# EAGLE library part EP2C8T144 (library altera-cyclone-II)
EP2C8T144 Auto generated by make-symbol-device-package-bsdl.ulp Rev. 19 Tip: Use split-device-symbol.ulp to generate a Device with multiple small symbols! Read HELP. Source: EP2C8T144.BSD
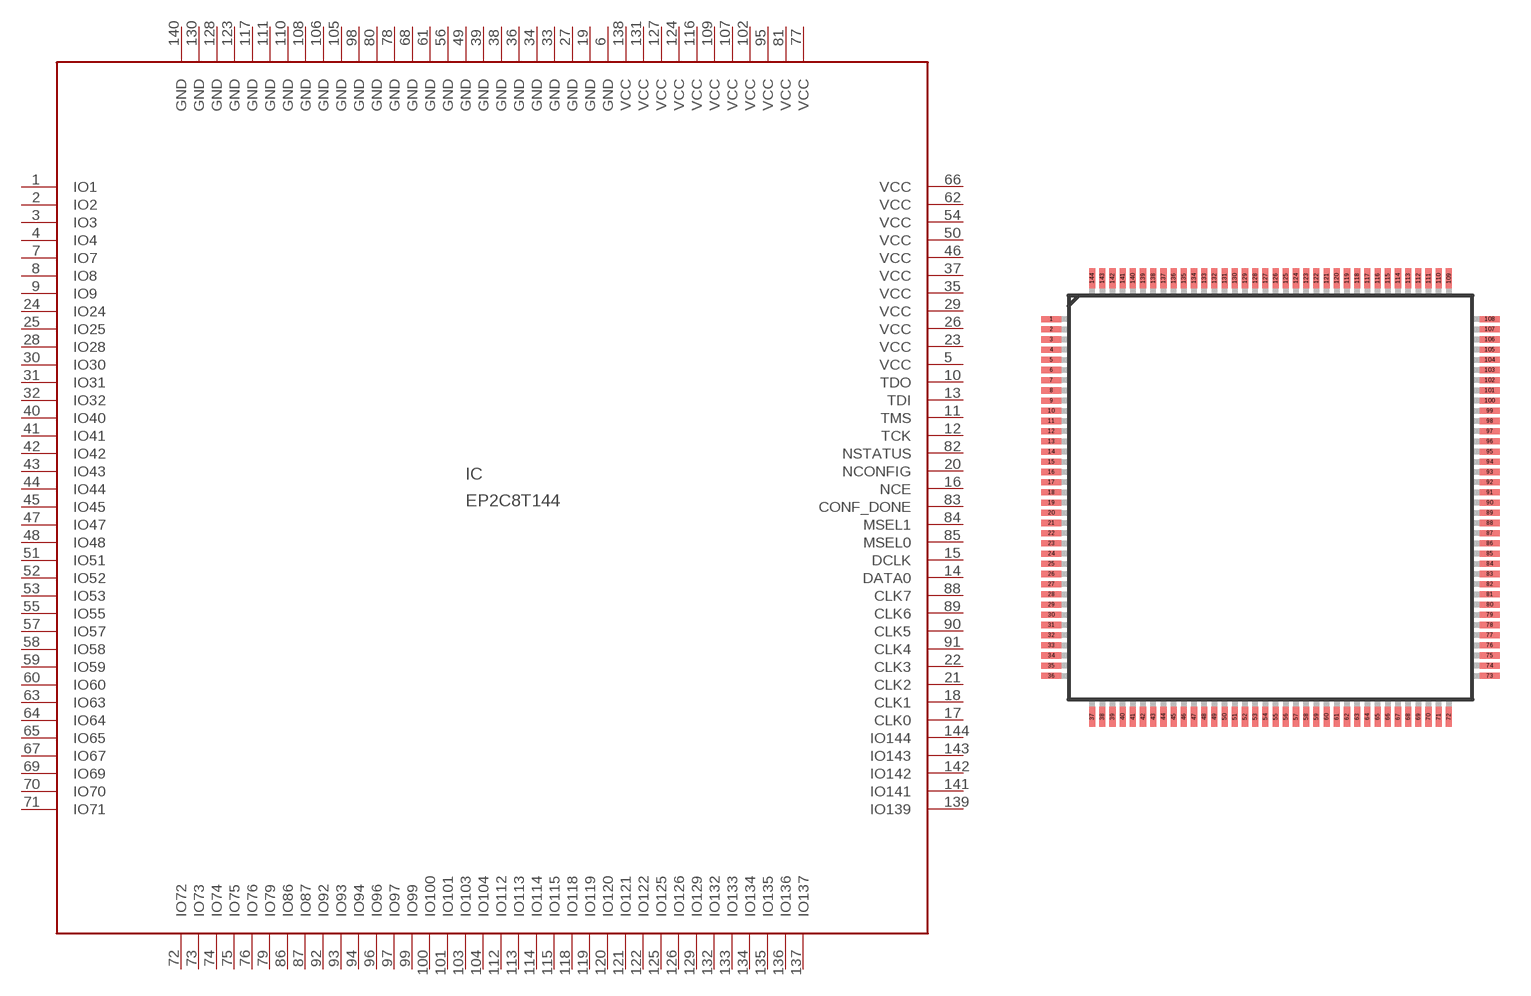
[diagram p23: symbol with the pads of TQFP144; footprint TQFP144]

Designator prefix IC

## EP2C8T144 (MPN: EP2C8T144C8N; OC_FARNELL: 1663192; OC_NEWARK: 51R0576)  [TQFP144]
1  IO1  out
2  IO2  out
3  IO3
4  IO4
5  VCC  pwr
6  GND  pwr
7  IO7
8  IO8
9  IO9
10  TDO  out
11  TMS  in
12  TCK  in
13  TDI  in
14  DATA0
15  DCLK
16  NCE  in
17  CLK0
18  CLK1
19  GND  pwr
20  NCONFIG  in
21  CLK2
22  CLK3
23  VCC  pwr
24  IO24
25  IO25
26  VCC  pwr
27  GND  pwr
28  IO28
29  VCC  pwr
30  IO30
31  IO31
32  IO32
33  GND  pwr
34  GND  pwr
35  VCC  pwr
36  GND  pwr
37  VCC  pwr
38  GND  pwr
39  GND  pwr
40  IO40
41  IO41
42  IO42
43  IO43
44  IO44
45  IO45
46  VCC  pwr
47  IO47
48  IO48
49  GND  pwr
50  VCC  pwr
51  IO51
52  IO52
53  IO53
54  VCC  pwr
55  IO55
56  GND  pwr
57  IO57
58  IO58
59  IO59
60  IO60
61  GND  pwr
62  VCC  pwr
63  IO63
64  IO64
65  IO65
66  VCC  pwr
67  IO67
68  GND  pwr
69  IO69
70  IO70
71  IO71
72  IO72
73  IO73
74  IO74
75  IO75
76  IO76
77  VCC  pwr
78  GND  pwr
79  IO79
80  GND  pwr
81  VCC  pwr
82  NSTATUS  in
83  CONF_DONE  in
84  MSEL1  in
85  MSEL0  in
86  IO86
87  IO87
88  CLK7
89  CLK6
90  CLK5
91  CLK4
92  IO92
93  IO93
94  IO94
95  VCC  pwr
96  IO96
97  IO97
98  GND  pwr
99  IO99
100  IO100
101  IO101
102  VCC  pwr
103  IO103
104  IO104
105  GND  pwr
106  GND  pwr
107  VCC  pwr
108  GND  pwr
109  VCC  pwr
110  GND  pwr
111  GND  pwr
112  IO112
113  IO113
114  IO114
115  IO115
116  VCC  pwr
117  GND  pwr
118  IO118
119  IO119
120  IO120
121  IO121
122  IO122
123  GND  pwr
124  VCC  pwr
125  IO125
126  IO126
127  VCC  pwr
128  GND  pwr
129  IO129
130  GND  pwr
131  VCC  pwr
132  IO132
133  IO133
134  IO134
135  IO135
136  IO136
137  IO137
138  VCC  pwr
139  IO139
140  GND  pwr
141  IO141
142  IO142
143  IO143
144  IO144

## Footprint TQFP144 (pad centres in mm)
TQFP144 Auto generated by make-symbol-device-package-bsdl.ulp Rev. 19
smd 1 x 0.3: 1 -10.75,8.75; 2 -10.75,8.25; 3 -10.75,7.75; 4 -10.75,7.25; 5 -10.75,6.75; 6 -10.75,6.25; 7 -10.75,5.75; 8 -10.75,5.25; 9 -10.75,4.75; 10 -10.75,4.25; 11 -10.75,3.75; 12 -10.75,3.25; 13 -10.75,2.75; 14 -10.75,2.25; 15 -10.75,1.75; 16 -10.75,1.25; 17 -10.75,0.75; 18 -10.75,0.25; 19 -10.75,-0.25; 20 -10.75,-0.75; 21 -10.75,-1.25; 22 -10.75,-1.75; 23 -10.75,-2.25; 24 -10.75,-2.75; 25 -10.75,-3.25; 26 -10.75,-3.75; 27 -10.75,-4.25; 28 -10.75,-4.75; 29 -10.75,-5.25; 30 -10.75,-5.75; 31 -10.75,-6.25; 32 -10.75,-6.75; 33 -10.75,-7.25; 34 -10.75,-7.75; 35 -10.75,-8.25; 36 -10.75,-8.75; 73 10.75,-8.75; 74 10.75,-8.25; 75 10.75,-7.75; 76 10.75,-7.25; 77 10.75,-6.75; 78 10.75,-6.25; 79 10.75,-5.75; 80 10.75,-5.25; 81 10.75,-4.75; 82 10.75,-4.25; 83 10.75,-3.75; 84 10.75,-3.25; 85 10.75,-2.75; 86 10.75,-2.25; 87 10.75,-1.75; 88 10.75,-1.25; 89 10.75,-0.75; 90 10.75,-0.25; 91 10.75,0.25; 92 10.75,0.75; 93 10.75,1.25; 94 10.75,1.75; 95 10.75,2.25; 96 10.75,2.75; 97 10.75,3.25; 98 10.75,3.75; 99 10.75,4.25; 100 10.75,4.75; 101 10.75,5.25; 102 10.75,5.75; 103 10.75,6.25; 104 10.75,6.75; 105 10.75,7.25; 106 10.75,7.75; 107 10.75,8.25; 108 10.75,8.75
smd 0.3 x 1: 37 -8.75,-10.75; 38 -8.25,-10.75; 39 -7.75,-10.75; 40 -7.25,-10.75; 41 -6.75,-10.75; 42 -6.25,-10.75; 43 -5.75,-10.75; 44 -5.25,-10.75; 45 -4.75,-10.75; 46 -4.25,-10.75; 47 -3.75,-10.75; 48 -3.25,-10.75; 49 -2.75,-10.75; 50 -2.25,-10.75; 51 -1.75,-10.75; 52 -1.25,-10.75; 53 -0.75,-10.75; 54 -0.25,-10.75; 55 0.25,-10.75; 56 0.75,-10.75; 57 1.25,-10.75; 58 1.75,-10.75; 59 2.25,-10.75; 60 2.75,-10.75; 61 3.25,-10.75; 62 3.75,-10.75; 63 4.25,-10.75; 64 4.75,-10.75; 65 5.25,-10.75; 66 5.75,-10.75; 67 6.25,-10.75; 68 6.75,-10.75; 69 7.25,-10.75; 70 7.75,-10.75; 71 8.25,-10.75; 72 8.75,-10.75; 109 8.75,10.75; 110 8.25,10.75; 111 7.75,10.75; 112 7.25,10.75; 113 6.75,10.75; 114 6.25,10.75; 115 5.75,10.75; 116 5.25,10.75; 117 4.75,10.75; 118 4.25,10.75; 119 3.75,10.75; 120 3.25,10.75; 121 2.75,10.75; 122 2.25,10.75; 123 1.75,10.75; 124 1.25,10.75; 125 0.75,10.75; 126 0.25,10.75; 127 -0.25,10.75; 128 -0.75,10.75; 129 -1.25,10.75; 130 -1.75,10.75; 131 -2.25,10.75; 132 -2.75,10.75; 133 -3.25,10.75; 134 -3.75,10.75; 135 -4.25,10.75; 136 -4.75,10.75; 137 -5.25,10.75; 138 -5.75,10.75; 139 -6.25,10.75; 140 -6.75,10.75; 141 -7.25,10.75; 142 -7.75,10.75; 143 -8.25,10.75; 144 -8.75,10.75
